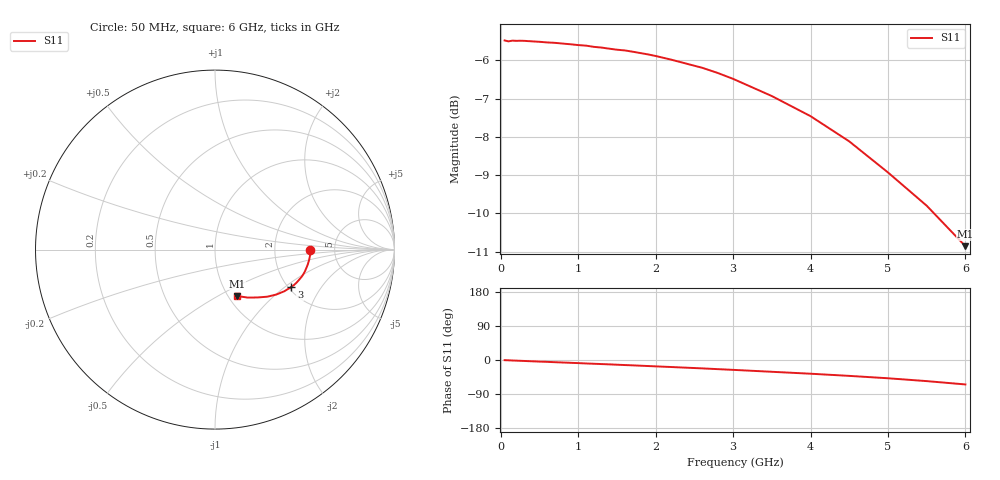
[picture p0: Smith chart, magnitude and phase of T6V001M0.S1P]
! SIEMENS Discrete & RF Semiconductors
! BAT62
! Si Schottky Diode in SOT143
! IF = 1 mA
! S-Parameters:  February  1997
# GHz  S  MA  R  50
!  f  S11
! GHz  MAG  ANG
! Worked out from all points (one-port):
!   34 points, 50 MHz to 6 GHz, reference 50 ohm
!   lowest |S11| = -10.9 dB at 6 GHz (marker M1), VSWR 1.80, Z = 54.9 - j31 ohm
!   |S11| at or under -10 dB: 5.596 GHz to end of sweep
!   S11 on the Smith chart (normalised r, x): 50 MHz: 3.27, -0.03; 3 GHz: 2.08, -1.11; 6 GHz: 1.10, -0.62
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0.05  0.5319 -0.4
0.1  0.5305 -0.8
0.15  0.5316 -1.3
0.3  0.5313 -2.5
0.4  0.5305 -3.4
0.5  0.5298 -4.2
0.6  0.5288 -4.9
0.7  0.5281 -5.8
0.8  0.527 -6.6
1  0.5246 -8.2
1.1  0.5237 -9.1
1.2  0.5218 -9.9
1.4  0.519 -11.5
1.6  0.5162 -13.3
1.7  0.5143 -14.1
1.8  0.5122 -15.0
2  0.5077 -16.8
2.2  0.5021 -18.5
2.4  0.496 -20.3
2.6  0.49 -22.1
2.8  0.4825 -24.1
3  0.4739 -26.0
3.5  0.4501 -31.1
4  0.4237 -36.2
4.5  0.3927 -41.9
5  0.3577 -48.2
5.5  0.3237 -55.7
6  0.2866 -64.5
